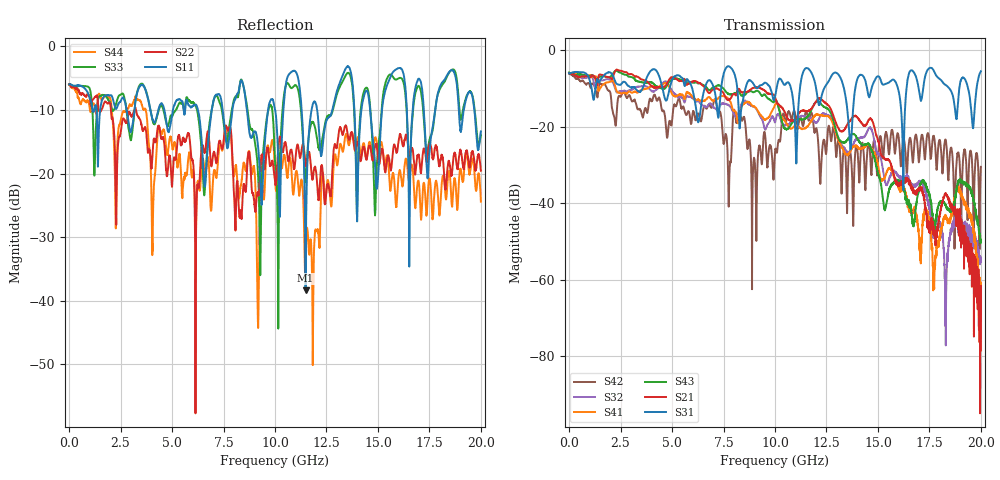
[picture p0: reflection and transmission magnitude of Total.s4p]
# Hz S RI R 50
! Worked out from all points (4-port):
!   20000 points, 1 MHz to 20 GHz, reference 50 ohm
!   strongest paths, dB at 1 MHz, 5.001 GHz, 10 GHz, 15 GHz, 20 GHz:
!     S31: -6.1, -7.9, -12.3, -6.9, -5.6
!     S21: -6.1, -7.1, -12.4, -23.6, -68.4
!     S43: -5.9, -7.6, -13.3, -32.1, -49.5
!     S41: -5.9, -11.5, -14.3, -29.9, -68.8
!     S32: -6.2, -10.6, -18.9, -27.0, -55.3
!     S42: -6.1, -18.6, -26.8, -29.5, -30.5
!   lowest |S11| = -38.4 dB at 11.48 GHz (marker M1), VSWR 1.02, Z = 49.3 - j0.947 ohm
!   |S11| at or under -10 dB: 6.26 GHz to 6.927 GHz (667.6 MHz wide, 10.1 % of centre); 8.639 GHz to 9.663 GHz (1.024 GHz wide, 11.2 % of centre); 12.05 GHz to 12.78 GHz (734.4 MHz wide, 5.92 % of centre)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
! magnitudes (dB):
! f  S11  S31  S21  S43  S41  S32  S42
! 1 MHz  -6.0  -6.1  -6.1  -5.9  -5.9  -6.2  -6.1
! 9.272 GHz  -20.0  -9.3  -9.9  -11.3  -16.8  -17.3  -25.4
! 10.95 GHz  -3.8  -17.6  -18.2  -18.4  -19.9  -18.4  -16.0
! 11.48 GHz  -38.4  -4.8  -15.9  -17.9  -20.3  -17.4  -16.3
! 17.72 GHz  -11.3  -5.5  -47.7  -46.6  -61.0  -48.1  -22.7
! 18.93 GHz  -10.3  -10.9  -45.5  -34.2  -36.4  -44.0  -27.6
! 20 GHz  -13.4  -5.6  -68.4  -49.5  -68.8  -55.3  -30.5
